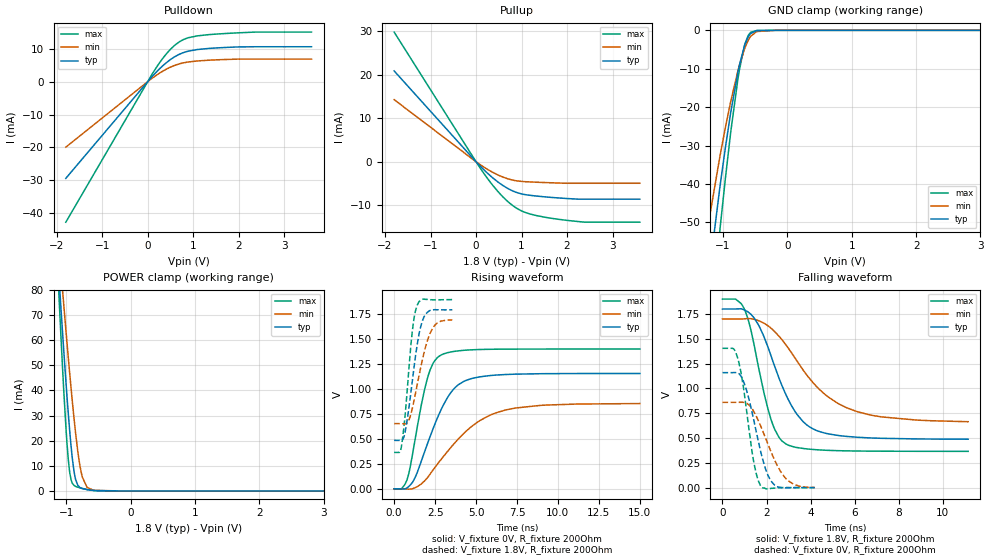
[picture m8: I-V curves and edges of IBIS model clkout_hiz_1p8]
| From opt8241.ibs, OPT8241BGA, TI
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|   clkout_hiz_1p8  Model
[Model]   clkout_hiz_1p8
Model_type   3-state
Polarity   Non-Inverting
Vmeas = 0.9
Vref  = 0
Cref  = 2pF
Rref  = 250
|   typ   min   max
|   (nom PVT)   (fast PVT)   (slow PVT)
C_comp   2.233e-12   2.012e-12   2.445e-12
| Where nom  PVT is Nominal Process, 1.8V, 27C
|   Fast PVT is Strong Process,  1.9V, -40C
|   Slow PVT is Weak Process,   1.7V, 125C
[Voltage Range]   1.8   1.7   1.9
|Junction Temperature
[Temperature Range]   27   125   -40
[Pullup Reference]   1.8   1.7   1.9
[Pulldown Reference]   0   0   0
[Power Clamp Reference]   1.8   1.7   1.9
[GND Clamp Reference]   0   0   0
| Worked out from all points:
|   slope of the pulldown table from 0 to 0.27 V, typ, clamps not added: 67 ohm
|   slope of the pullup table from 0 to 0.27 V, typ, clamps not added: 96 ohm
|   GND clamp passes 1 mA (typ) near -0.58 V on its own axis
|   POWER clamp passes 1 mA (typ) near -0.76 V on its own axis
|   falling waveform, V_fixture 1.8V, R_fixture 200Ohm: 20-80 % time 1.49ns typ, 2.4ns min, 941ps max; typ from 1.8 V to 0.488 V
|   rising waveform, V_fixture 0V, R_fixture 200Ohm: 20-80 % time 1.74ns typ, 2.93ns min, 1.01ns max; typ from 0 V to 1.16 V
|   rising waveform, V_fixture 1.8V, R_fixture 200Ohm: 20-80 % time 653ps typ, 845ps min, 488ps max; typ from 0.486 V to 1.8 V
|   falling waveform, V_fixture 0V, R_fixture 200Ohm: 20-80 % time 735ps typ, 1.01ns min, 532ps max; typ from 1.16 V to 0.001 V
[Pulldown]
|   Voltage   I(typ)   I(min)   I(max)
-1.8V     -29.39mA   -19.91mA   -42.7mA
113.3mV   1.797mA    1.196mA    2.645mA
360mV     5.171mA    3.414mA    7.591mA
489.9mV   6.607mA    4.338mA    9.677mA
605.4mV   7.655mA    4.999mA    11.18mA
778.3mV   8.786mA    5.686mA    12.74mA
898mV     9.277mA    5.978mA    13.35mA
1.329V    10.07mA    6.498mA    14.26mA
2.342V    10.6mA     6.839mA    15.04mA
3.598V    10.6mA     6.839mA    15.05mA
[GND Clamp]
|   Voltage   I(typ)   I(min)   I(max)
-1.8V     -241.9mA   -138.2mA   -348.9mA
-1.295V   -73.8mA    -56.93mA   -94.29mA
-1.049V   -40.84mA   -32.87mA   -52.02mA
-1.042V   -39.89mA   -32.18mA   -50.79mA
-885.6mV  -21.89mA   -18.9mA    -27.16mA
-768.1mV  -10.82mA   -10.47mA   -12.55mA
-663.8mV  -3.855mA   -4.706mA   -3.708mA
-611.7mV  -1.779mA   -2.684mA   -1.411mA
-568.8mV  -794.1uA   -1.514mA   -509.6uA
-477.4mV  -89.94uA   -315uA     -33.24uA
-180mV    0A         -253.3nA   0A
3.6V      0A         0A         0A
[Pullup]
|   Voltage   I(typ)   I(min)   I(max)
-1.8V     20.9mA     14.29mA    29.83mA
113.4mV   -1.24mA    -829uA     -1.798mA
306.3mV   -3.156mA   -2.085mA   -4.605mA
467.8mV   -4.549mA   -2.969mA   -6.686mA
597mV     -5.506mA   -3.551mA   -8.148mA
792mV     -6.644mA   -4.19mA    -9.965mA
909.4mV   -7.129mA   -4.42mA    -10.8mA
1.114V    -7.619mA   -4.607mA   -11.79mA
1.329V    -7.897mA   -4.713mA   -12.39mA
1.761V    -8.292mA   -4.879mA   -13.17mA
2.382V    -8.614mA   -4.95mA    -13.89mA
3.6V      -8.614mA   -4.95mA    -13.91mA
[POWER Clamp]
|   Voltage   I(typ)   I(min)   I(max)
-1.8V     371.7mA    319.2mA    464.8mA
-1.115V   84.75mA    97.02mA    77.29mA
-1.086V   73.09mA    87.82mA    61.92mA
-1.048V   58.36mA    76.06mA    43.04mA
-971.6mV  31.12mA    53.36mA    12.8mA
-929.8mV  18.46mA    41.55mA    4.733mA
-870.1mV  6.114mA    26.09mA    1.986mA
-822.6mV  2.259mA    15.67mA    1.478mA
-756.2mV  960.3uA    5.742mA    1.007mA
-679.7mV  528.4uA    1.426mA    564.7uA
-585.9mV  212.9uA    346.8uA    184.6uA
3.6V      0A         0A         0A
[Ramp]
R_load = 200
|   typ   min   max
dV/dt_r   0.694451/1.73935e-09   0.513445/2.93356e-09   0.841715/1.00636e-09
dV/dt_f   0.787572/1.49552e-09   0.625278/2.41925e-09   0.920475/9.40268e-10
[Falling Waveform]
V_fixture = 1.8V
V_fixture_min = 1.7V
V_fixture_max = 1.9V
R_fixture = 200Ohm
|   Time   V(typ)   V(min)   V(max)
0s        1.8V       1.7V       1.9V
594ps     1.8V       1.7V       1.9V
1.016ns   1.789V     1.701V     1.789V
1.274ns   1.751V     1.703V     1.605V
1.608ns   1.651V     1.685V     1.245V
2.2ns     1.332V     1.608V     690.4mV
2.884ns   936.1mV    1.438V     440.6mV
3.95ns    613.1mV    1.101V     388.1mV
5.646ns   516.4mV    804.9mV    370.9mV
11.16ns   488.4mV    664.6mV    366.2mV
[Rising Waveform]
V_fixture = 0V
V_fixture_min = 0V
V_fixture_max = 0V
R_fixture = 200Ohm
|   Time   V(typ)   V(min)   V(max)
0s        772.9pV    49.28nV    368.1pV
448ps     -1.2mV     231.4uV    1.209mV
786ps     9.616mV    -2.276mV   90.83mV
1.266ns   108.5mV    10.09mV    482.7mV
2ns       436.7mV    105.4mV    1.09V
2.382ns   605.5mV    189.9mV    1.261V
2.88ns    799.4mV    297.8mV    1.344V
4.27ns    1.08V      559.4mV    1.39V
6.798ns   1.147V     790.7mV    1.402V
15ns      1.157V     855.7mV    1.403V
[Rising Waveform]
V_fixture = 1.8V
V_fixture_min = 1.7V
V_fixture_max = 1.9V
R_fixture = 200Ohm
|   Time   V(typ)   V(min)   V(max)
0s        486.2mV    654.2mV    364.9mV
330ps     485.6mV    654.4mV    365.6mV
438ps     485.1mV    653.8mV    417.9mV
690ps     588.5mV    652.3mV    775.7mV
1.1ns     1.068V     799.3mV    1.567V
1.234ns   1.243V     901.8mV    1.729V
1.418ns   1.457V     1.053V     1.846V
1.81ns    1.72V      1.355V     1.904V
2.376ns   1.796V     1.618V     1.897V
3.55ns    1.796V     1.695V     1.899V
[Falling Waveform]
V_fixture = 0V
V_fixture_min = 0V
V_fixture_max = 0V
R_fixture = 200Ohm
|   Time   V(typ)   V(min)   V(max)
0s        1.159V     859.7mV    1.404V
496ps     1.159V     859.7mV    1.4V
698ps     1.156V     859.8mV    1.3V
1.006ns   1.04V      857.7mV    924.7mV
1.402ns   701.8mV    774.9mV    281.2mV
1.73ns    368.5mV    623.8mV    20.44mV
2.08ns    117.8mV    430.8mV    -14.83mV
2.462ns   11.75mV    233.9mV    -1.954mV
3.22ns    456.7uV    35.94mV    1.018mV
4.184ns   990.6uV    1.935mV    200.2uV
